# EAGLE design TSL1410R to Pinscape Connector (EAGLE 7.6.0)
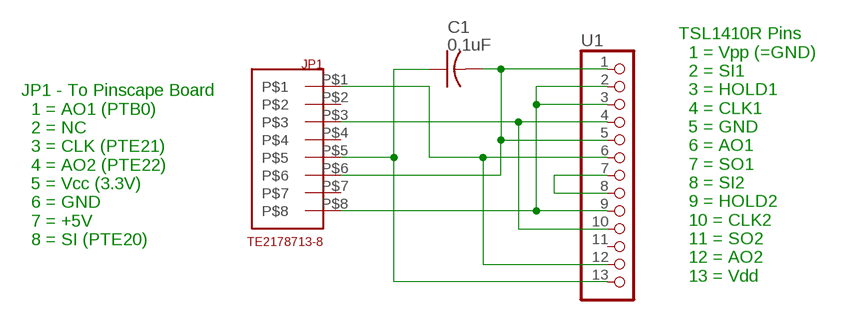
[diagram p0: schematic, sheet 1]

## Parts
C1  0.1uF  C-US025-024X044  [C025-024X044]
JP1  TE2178713-8  [IDC-PADDLE-8]
U1  PINHD-1X13  [1X13]

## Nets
GND: C1.2 JP1.P$6 U1.1 U1.5
N$1: JP1.P$8 U1.2 U1.3 U1.9
N$2: U1.7 U1.8
N$3: JP1.P$3 U1.4 U1.10
N$5: JP1.P$1 U1.6 U1.12
N$9: C1.1 JP1.P$5 U1.13
Unconnected: JP1.P$2 JP1.P$4 JP1.P$7 U1.11

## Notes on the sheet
- JP1 - To Pinscape Board
    1 = AO1 (PTB0)
    2 = NC
    3 = CLK (PTE21)
    4 = AO2 (PTE22)
    5 = Vcc (3.3V)
    6 = GND
    7 = +5V
    8 = SI (PTE20)
- TSL1410R Pins
    1 = Vpp (=GND)
    2 = SI1
    3 = HOLD1
    4 = CLK1
    5 = GND
    6 = AO1
    7 = SO1
    8 = SI2
    9 = HOLD2
    10 = CLK2
    11 = SO2
    12 = AO2
    13 = Vdd

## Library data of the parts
C1 = rcl:C-US: CAPACITOR, American symbol
JP1 = TEConnectivity:TE2178713-8
U1 = pinhead:PINHD-1X13: PIN HEADER

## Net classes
0 default: width 0.254 mm, drill 0.254 mm, clearance 0.254 mm

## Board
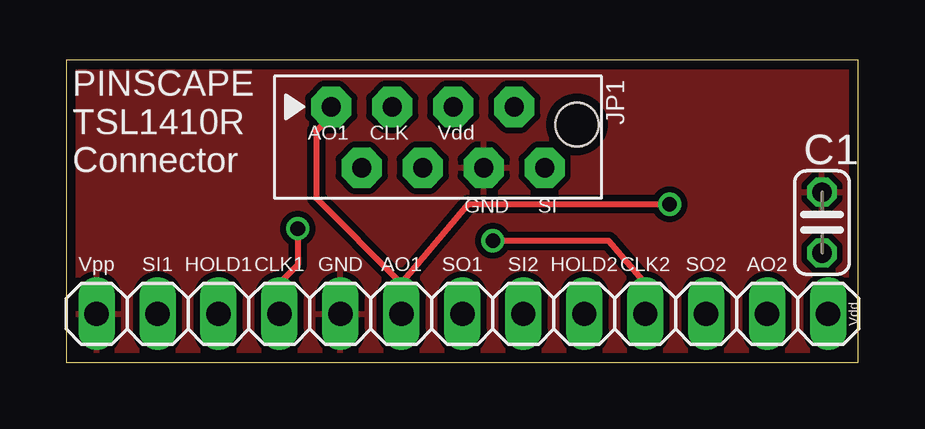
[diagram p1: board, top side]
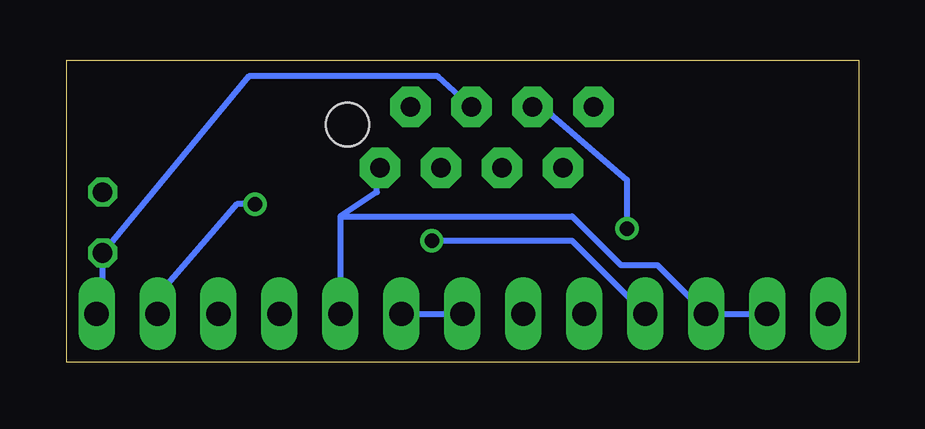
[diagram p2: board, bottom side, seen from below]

Size 33 x 12.62 mm. Coordinates in mm from the lower left corner, seen from the top.
Outline: 0,0 33,0 33,12.62 0,12.62 0,0
Copper layers (1*16): Top 0.0356mm / dielectric 1.5011mm / Bottom 0.0356mm
Design rules "OSH Park": minimum track width 6mil, minimum drill 13mil, track to track 6mil, track to pad 6mil, pad to pad 6mil, via to via 6mil, smd to smd 6mil, copper to edge 15mil, drill to drill 6mil, minimum pad ring 7mil, minimum via ring 7mil, stop-mask expansion 3mil, vias tented up to drill 0mil, thermal gap 10mil

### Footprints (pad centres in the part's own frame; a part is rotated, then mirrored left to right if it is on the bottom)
C025-024X044 = drill 0.813 octagon: 1 -1.27,0; 2 1.27,0
IDC-PADDLE-8 = drill 0.8 pad 1.676 octagon: P$1 -4.445,1.27; P$2 -3.175,-1.27; P$3 -1.905,1.27; P$4 -0.635,-1.27; P$5 0.635,1.27; P$6 1.905,-1.27; P$7 3.175,1.27; P$8 4.445,-1.27 | hole 1.8: 5.795,0.53
1X13 = drill 1.016 long: 1 -15.24,0; 2 -12.7,0; 3 -10.16,0; 4 -7.62,0; 5 -5.08,0; 6 -2.54,0; 7 0,0; 8 2.54,0; 9 5.08,0; 10 7.62,0; 11 10.16,0; 12 12.7,0; 13 15.24,0

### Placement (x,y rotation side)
C1  31.5,5.84 90 top
JP1  15.49,9.4 0 top
U1  16.51,2.03 0 top

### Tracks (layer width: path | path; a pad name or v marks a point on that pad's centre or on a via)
GND
  pour Top: 0,12.45 33.02,12.45 33.02,0.25 0,0.25
N$1
  Bottom 0.254: U1.2 U1.3 8.38,4.06 9.91,4.06 11.94,6.1 21.59,6.1 | 21.59,6.1 U1.9 | 21.59,6.1 20.07,7.11 20.07,8.13 JP1.P$8
N$2
  Bottom 0.254: U1.8 U1.7
N$3  (via drill 0.61)
  Top 0.254: U1.4 8.89,3.3 9.65,4.06 v9.65,5.59 | U1.10 24.13,3.3 22.61,5.08 v17.78,5.08
  Bottom 0.254: JP1.P$3 13.21,10.67 9.65,7.62 v9.65,5.59 | v17.78,5.08 11.94,5.08 U1.4
N$5  (via drill 0.61)
  Top 0.254: 13.97,3.3 U1.6 | 13.97,3.3 10.41,6.86 10.41,9.65 10.92,10.16 10.92,10.92 JP1.P$1 | v25.15,6.6 16.76,6.6 13.97,3.3
  Bottom 0.254: v25.15,6.6 25.91,6.6 29.21,2.79 U1.12
N$9
  Bottom 0.254: U1.13 31.5,2.29 C1.1 25.4,11.94 17.53,11.94 JP1.P$5

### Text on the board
tNames: PINSCAPE / TSL1410R / Connector | AO1 | CLK | Vdd | GND | SI | Vpp | SI1 | HOLD1 | CLK1 | GND | AO1 | SO1 | SI2 | HOLD2 | CLK2 | SO2 | AO2 | Vdd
